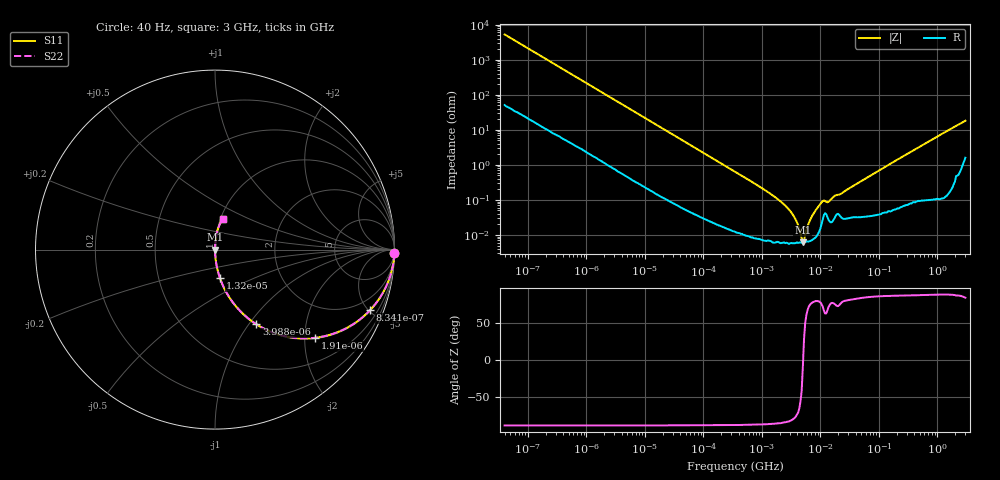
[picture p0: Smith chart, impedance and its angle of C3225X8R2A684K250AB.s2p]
! S-parameter Generated by TDK Corporation
! Copyright(C) 2015 TDK Corporation.
! All Rights Reserved.
! TDK P/N: C3225X8R2A684K250AB (Multilayer Ceramic Chip Capacitors)
! Property: C=680nF
! Size(LxWxT): 3.2x2.5x2.5mm, 0.126x0.098x0.098inches
! Model Type: s2p (Touchstone File Format Version 1.0)
! Frequency: DC=Yes Start=0.00004MHz Stop=3000MHz 396points Log-sweep
! Note: This model was converted from impedance.
! Model Generated on Jun. 23, 2015
! Hash(MD5):
! Port Assignments:
!  1 ---| |--- 2
! Applicable Conditions:
!  Temperature = 25 degC
!  DC Bias Voltage = 0 V
!  Small Signal Operation
! Terms and conditions regarding TDK Simulation Models
! (1)This simulation model is being provided solely for informational purposes. Please refer to the specifications of the products in terms of detailed characteristics of such products.
! (2)In no event shall TDK Corporation of any of its subsidiaries be liable for any loss or damage arising, directly or indirectly,
!  From any information contained in this simulation model, including, but not limited to loss or damages arising from any inaccuracies, omissions or errors in connection with such information.
! (3)Any and all copyrights on this simulation model are owned by TDK Corporation.
!  Duplication or redistribution of this simulation model without prior written permission from TDK Corporation is prohibited.
! (4)This simulation model is subject to any modification or change without any prior notice.
! (5)Neither TDK Corporation nor any of its subsidiaries shall make any warranty, express or implied,
!  Including but not limited to the correctness, implied warranties of merchantability and fitness for a particular purpose with respect to this simulation models.
! (6)The use of this simulation model shall be deemed to have consented to the terms and conditions hereof.
# MHz S MA R 50
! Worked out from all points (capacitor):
!   395 points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, 40 Hz to 3 GHz, reference 50 ohm
!   read as one part in series: C = 759 nF near 41.88 Hz
!   lowest |Z| = 6.23 mohm at 4.999 MHz (marker M1)
!   series resonance near 5.059 MHz, so ESL is about 1.3 nH
!   S11 on the Smith chart (normalised r, x): 40 Hz: open; 834.1 Hz: 1.06, -5.13; 1.91 kHz: 1.02, -2.25; 3.988 kHz: 1.01, -1.08; 13.2 kHz: 1.00, -0.33; 3 GHz: 1.03, +0.36
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4e-05  0.9996 -1.1  0.01917 88.3  0.01917 88.3  0.9996 -1.1
0.0002299237  0.9931 -6.2  0.1077 83.2  0.1077 83.2  0.9931 -6.2
0.000834128  0.9282 -21.2  0.362 68.1  0.362 68.1  0.9282 -21.2
0.001909884  0.744 -41.3  0.6603 48.1  0.6603 48.1  0.744 -41.3
0.003988472  0.4746 -61.1  0.8752 28.3  0.8752 28.3  0.4746 -61.1
0.01319716  0.1628 -80.0  0.9849 9.4  0.9849 9.4  0.1628 -80.0
0.01739424  0.1245 -82.2  0.9909 7.2  0.9909 7.2  0.1245 -82.2
0.3464102  0.006422 -88.5  0.9999 0.4  0.9999 0.4  0.006422 -88.5
1.37789  0.001524 -87.4  0.9999 0.1  0.9999 0.1  0.001524 -87.4
2.506407  0.0006902 -85.1  0.9999 0.0  0.9999 0.0  0.0006902 -85.1
3.459106  0.0003554 -80.5  0.9999 0.0  0.9999 0.0  0.0003554 -80.5
3.971241  0.0002293 -74.4  0.9999 0.0  0.9999 0.0  0.0002293 -74.4
4.5592  0.0001124 -56.6  0.9999 0.0  0.9999 0.0  0.0001124 -56.6
4.998775  6.229e-05 -10.2  0.9999 0.0  0.9999 0.0  6.229e-05 -10.2
5.480732  9.757e-05 49.9  0.9999 -0.0  0.9999 -0.0  9.757e-05 49.9
6.292177  0.0002152 72.5  0.9999 -0.0  0.9999 -0.0  0.0002152 72.5
7.22376  0.000353 78.2  0.9999 -0.0  0.9999 -0.0  0.000353 78.2
10.93076  0.0009223 72.6  0.9997 -0.1  0.9997 -0.1  0.0009223 72.6
13.75903  0.0008888 72.3  0.9997 -0.0  0.9997 -0.0  0.0008888 72.3
18.13479  0.001351 75.1  0.9997 -0.1  0.9997 -0.1  0.001351 75.1
150.6385  0.01033 86.7  0.9995 -0.6  0.9995 -0.6  0.01033 86.7
3000  0.1755 74.9  0.9691 -10.1  0.9691 -10.1  0.1755 74.9
